{attribute 'qualified_only'}
TYPE E_AdsWriteState :
(
    Idle,
    StartGetHandle,
    WaitGetHandle,
    StartWriteValue,
    WaitWriteValue,
    StartReleaseHandle,
    WaitReleaseHandle
);
END_TYPE
